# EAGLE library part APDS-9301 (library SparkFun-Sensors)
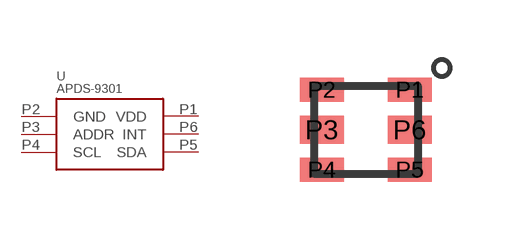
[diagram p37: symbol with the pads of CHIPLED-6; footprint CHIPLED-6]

Designator prefix U

## APDS-9301 (PROD_ID: IC-13662; VALUE: APDS-9301)  [CHIPLED-6]
P1  VDD
P2  GND
P3  ADDR
P4  SCL
P5  SDA
P6  INT

## Footprint CHIPLED-6 (pad centres in mm)
CHIPLED-6 package Used by APDS-9301
smd 1.1 x 0.6: P1 1.1,1; P2 -1.1,1; P4 -1.1,-1; P5 1.1,-1
smd 1.1 x 0.7: P3 -1.1,0; P6 1.1,0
